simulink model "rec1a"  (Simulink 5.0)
settings: Solver=ode15s  StartTime=0.0  StopTime=0.05  MaxStep=1e-4  RelTol=1e-5  AbsTol=1e-5

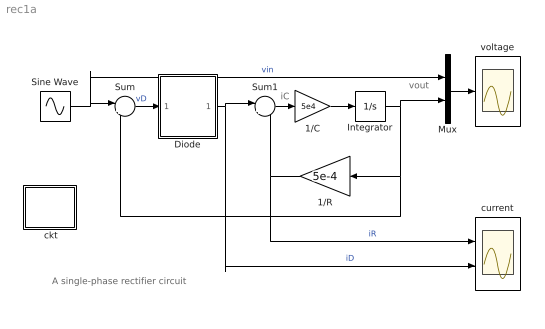
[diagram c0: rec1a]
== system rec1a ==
  note: vout
  note: A single-phase rectifier circuit
  note: iC
  " ckt" : Subsystem
  1/C : Gain  Gain=5e4
  1/R : Gain  Orientation=left  Gain=5e-4
  Diode : Subsystem
  Integrator : Integrator
  Mux : Mux  Inputs=2
  Sine Wave : Sin  Amplitude=24  Frequency=2*pi*60  SampleTime=0
  Sum : Sum  Inputs=|+-
  Sum1 : Sum  Inputs=|+-
  current : Scope  NumInputPorts=2
  voltage : Scope
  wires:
  1/C/1 -> Integrator/1
  Integrator/1 -> 1/R/1, Sum/2, Mux/2
  Mux/1 -> voltage/1
  Sine Wave/1 -> Sum/1, Mux/1  "vin"
  1/R/1 -> Sum1/2, current/1  "iR"
  Diode/1(iD) -> Sum1/1, current/2  "iD"
  Sum1/1 -> 1/C/1
  Sum/1 -> Diode/1(vD)  "vD"

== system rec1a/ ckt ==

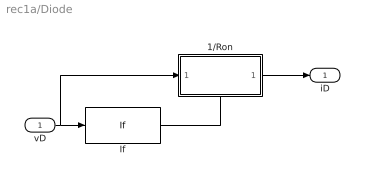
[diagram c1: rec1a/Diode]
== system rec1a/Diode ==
  vD : Inport
  1/Ron : Subsystem  TreatAsAtomicUnit=on
  If : If  IfExpression=u1>=0  ShowElse=off
  iD : Outport
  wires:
  vD/1 -> If/1, 1/Ron/1(a)
  1/Ron/1(b) -> iD/1
  If/1 -> 1/Ron/Action

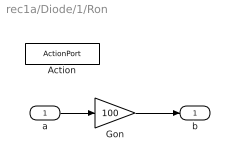
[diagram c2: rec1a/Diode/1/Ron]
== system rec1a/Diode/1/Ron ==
  a : Inport
  Action : ActionPort  InitializeStates=reset  ActionType=then
  Gon : Gain  Gain=100
  b : Outport  OutputWhenDisabled=reset  InitialOutput=0
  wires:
  a/1 -> Gon/1
  Gon/1 -> b/1
